// TwinCAT 3 PLC project TC3_SortingSystem_Simu
// libraries:
//   Tc2_Standard, * (Beckhoff Automation GmbH)
//   Tc2_System, * (Beckhoff Automation GmbH)
//   Tc3_Interfaces, * (Beckhoff Automation GmbH)
//   Tc3_Module, * (Beckhoff Automation GmbH)
// project tree:
//   / PlcTask_Simu.TcTTO, Visualization Manager.TcVMO
//   POUs/ MAIN_Simu.TcPOU
// real-time tasks:
//   TASK PlcTask: cycle T#10ms, priority 20, ADS port 350
//   TASK PlcTask_Simu: cycle T#10ms, priority 21, ADS port 351
// motion (NC):
//   TASK NC-Task 1 SAF: cycle T#2ms, priority 4, ADS port 501
//   TASK NC-Task 1 SVB: cycle T#10ms, priority 8, ADS port 511
//   AXIS Axis MetalSorting (id 1)
//     OtherSettings: AllowMotionCmdToSlave=true
//     encoder EncType=1
//     drive DrvType=5
//       TimeComp: TaskDelayCycles=1
//     controller CtrType=1
//       CtrPara: PriorControlFactor=1
//         Observer: BandWidth=20
//   AXIS Axis PlasticSorting (id 2)
//     OtherSettings: AllowMotionCmdToSlave=true
//     encoder EncType=1
//     drive DrvType=5
//     controller CtrType=1
//       CtrPara: PriorControlFactor=1
//         Observer: BandWidth=20
//   AXIS Axis Separating (id 3)
//     OtherSettings: AllowMotionCmdToSlave=true
//     encoder EncType=1
//     drive DrvType=5
//       TimeComp: TaskDelayCycles=1
//     controller CtrType=1
//       CtrPara: PriorControlFactor=1
//         Observer: BandWidth=20
// variable links:
//   TC3_SortingSystem_PLC/TC3_SortingSystem_PLC Instance <-> NC-Task 1 SAF/Axes/Axis MetalSorting
//     PlcTask Outputs/MAIN.fbMetalSorting.fbAxis.AxisRef.PlcToNc <-> Inputs/Axis MetalSorting_FromPlc
//     PlcTask Inputs/MAIN.fbMetalSorting.fbAxis.AxisRef.NcToPlc <-> Outputs/Axis MetalSorting_ToPlc
//   TC3_SortingSystem_PLC/TC3_SortingSystem_PLC Instance <-> NC-Task 1 SAF/Axes/Axis PlasticSorting
//     PlcTask Outputs/MAIN.fbPlasticSorting.fbAxis.AxisRef.PlcToNc <-> Inputs/Axis PlasticSorting_FromPlc
//     PlcTask Inputs/MAIN.fbPlasticSorting.fbAxis.AxisRef.NcToPlc <-> Outputs/Axis PlasticSorting_ToPlc
//   TC3_SortingSystem_PLC/TC3_SortingSystem_PLC Instance <-> NC-Task 1 SAF/Axes/Axis Separating
//     PlcTask Outputs/MAIN.fbSeparateModule.fbAxis.AxisRef.PlcToNc <-> Inputs/Axis Separating_FromPlc
//     PlcTask Inputs/MAIN.fbSeparateModule.fbAxis.AxisRef.NcToPlc <-> Outputs/Axis Separating_ToPlc
//   TC3_SortingSystem_PLC/TC3_SortingSystem_PLC Instance <-> TC3_SortingSystem_Simu/TC3_SortingSystem_Simu Instance
//     PlcTask Inputs/MAIN.fbSeparateModule.fbClampTemp.lrTempCurrent <-> PlcTask_Simu Outputs/MAIN_Simu.lrClampTempCurrent
//     PlcTask Inputs/MAIN.fbSeparateModule.fbClampTempDiag.bAtWorkPos <-> PlcTask_Simu Outputs/MAIN_Simu.bClampAtWork
//     PlcTask Inputs/MAIN.fbSeparateModule.fbClampTempDiag.lrTempMax <-> PlcTask_Simu Outputs/MAIN_Simu.lrClampTempMax
//     PlcTask Inputs/MAIN.fbSeparateModule.fbClampTempRecord.bAtBasePos <-> PlcTask_Simu Outputs/MAIN_Simu.bClampAtBase
//     PlcTask Inputs/MAIN.fbSeparateModule.fbClampTempRecord.lrTempCurrent <-> PlcTask_Simu Outputs/MAIN_Simu.lrClampTempCurrent
//     PlcTask Inputs/MAIN.fbSeparateModule.fbBarrier.bAtWorkPos <-> PlcTask_Simu Outputs/MAIN_Simu.bBarrierAtWork
//     PlcTask Inputs/MAIN.fbSeparateModule.fbBarrierDiag.bAtWorkPos <-> PlcTask_Simu Outputs/MAIN_Simu.bBarrierAtWork
//     PlcTask Inputs/MAIN.fbSeparateModule.fbBarrierTemp.bAtWorkPos <-> PlcTask_Simu Outputs/MAIN_Simu.bBarrierAtWork
//     PlcTask Inputs/MAIN.fbSeparateModule.fbBarrierTempDiag.bAtBasePos <-> PlcTask_Simu Outputs/MAIN_Simu.bBarrierAtBase
//     PlcTask Inputs/MAIN.fbSeparateModule.fbBarrierTempDiag.lrTempCurrent <-> PlcTask_Simu Outputs/MAIN_Simu.lrBarrierTemp
//     PlcTask Inputs/MAIN.fbMetalSorting.fbCylinder.bAtBasePos <-> PlcTask_Simu Outputs/MAIN_Simu.bMetalAtBase
//     PlcTask Inputs/MAIN.fbMetalSorting.fbCylinderDiag.bAtBasePos <-> PlcTask_Simu Outputs/MAIN_Simu.bMetalAtBase
//     PlcTask Inputs/MAIN.fbSeparateModule.fbBarrierTempRecord.bAtWorkPos <-> PlcTask_Simu Outputs/MAIN_Simu.bBarrierAtWork
//     PlcTask Inputs/MAIN.fbMetalSorting.fbCylinderTemp.bAtBasePos <-> PlcTask_Simu Outputs/MAIN_Simu.bMetalAtBase
//     PlcTask Outputs/MAIN.fbVisu.lrYClamp <-> PlcTask_Simu Inputs/MAIN_Simu.lrYClamp
//     PlcTask Outputs/MAIN.fbVisu.lrYBarrier <-> PlcTask_Simu Inputs/MAIN_Simu.lrYBarrier
//     PlcTask Outputs/MAIN.fbVisu.lrYMetal <-> PlcTask_Simu Inputs/MAIN_Simu.lrYMetal
//     PlcTask Outputs/MAIN.fbVisu.lrYPlastic <-> PlcTask_Simu Inputs/MAIN_Simu.lrYPlastic
//     PlcTask Inputs/MAIN.fbMetalSorting.fbCylinderTempDiag.bAtWorkPos <-> PlcTask_Simu Outputs/MAIN_Simu.bMetalAtWork
//     PlcTask Outputs/MAIN.fbVisu.lrBoxX <-> PlcTask_Simu Inputs/MAIN_Simu.lrBoxX
//     PlcTask Inputs/MAIN.fbPlasticSorting.fbSensorDelay.bInput <-> PlcTask_Simu Outputs/MAIN_Simu.bPlasticSensor
//     PlcTask Inputs/MAIN.fbPlasticSorting.fbCylinder.bAtWorkPos <-> PlcTask_Simu Outputs/MAIN_Simu.bPlasticAtWork
//     PlcTask Inputs/MAIN.fbMetalSorting.fbCylinderTempRecord.bAtBasePos <-> PlcTask_Simu Outputs/MAIN_Simu.bMetalAtBase
//     PlcTask Inputs/MAIN.fbPlasticSorting.fbCylinderDiag.bAtWorkPos <-> PlcTask_Simu Outputs/MAIN_Simu.bPlasticAtWork
//     PlcTask Outputs/MAIN.fbVisu.lrBoxY <-> PlcTask_Simu Inputs/MAIN_Simu.lrBoxY
//     PlcTask Inputs/MAIN.fbPlasticSorting.fbCylinderTemp.bAtWorkPos <-> PlcTask_Simu Outputs/MAIN_Simu.bPlasticAtWork
//     PlcTask Inputs/MAIN.fbPlasticSorting.fbCylinderTempDiag.bAtBasePos <-> PlcTask_Simu Outputs/MAIN_Simu.bPlasticAtBase
//     PlcTask Inputs/MAIN.fbSeparateModule.fbClamp.bAtBasePos <-> PlcTask_Simu Outputs/MAIN_Simu.bClampAtBase
//     PlcTask Inputs/MAIN.fbSeparateModule.fbClampDiag.bAtBasePos <-> PlcTask_Simu Outputs/MAIN_Simu.bClampAtBase
//     PlcTask Inputs/MAIN.fbSeparateModule.fbClampTemp.bAtBasePos <-> PlcTask_Simu Outputs/MAIN_Simu.bClampAtBase
//     PlcTask Inputs/MAIN.fbSeparateModule.fbClampTempDiag.bAtBasePos <-> PlcTask_Simu Outputs/MAIN_Simu.bClampAtBase
//     PlcTask Inputs/MAIN.fbSeparateModule.fbBarrier.bAtBasePos <-> PlcTask_Simu Outputs/MAIN_Simu.bBarrierAtBase
//     PlcTask Inputs/MAIN.fbSeparateModule.fbBarrierDiag.bAtBasePos <-> PlcTask_Simu Outputs/MAIN_Simu.bBarrierAtBase
//     PlcTask Inputs/MAIN.fbSeparateModule.fbBarrierTemp.bAtBasePos <-> PlcTask_Simu Outputs/MAIN_Simu.bBarrierAtBase
//     PlcTask Inputs/MAIN.fbSeparateModule.fbBarrierTempRecord.bAtBasePos <-> PlcTask_Simu Outputs/MAIN_Simu.bBarrierAtBase
//     PlcTask Inputs/MAIN.fbMetalSorting.fbCylinderTempDiag.bAtBasePos <-> PlcTask_Simu Outputs/MAIN_Simu.bMetalAtBase
//     PlcTask Inputs/MAIN.fbPlasticSorting.fbCylinderTempRecord.bAtWorkPos <-> PlcTask_Simu Outputs/MAIN_Simu.bPlasticAtWork
//     PlcTask Inputs/MAIN.fbPlasticSorting.fbCylinder.bAtBasePos <-> PlcTask_Simu Outputs/MAIN_Simu.bPlasticAtBase
//     PlcTask Inputs/MAIN.fbPlasticSorting.fbCylinderDiag.bAtBasePos <-> PlcTask_Simu Outputs/MAIN_Simu.bPlasticAtBase
//     PlcTask Inputs/MAIN.fbPlasticSorting.fbCylinderTemp.bAtBasePos <-> PlcTask_Simu Outputs/MAIN_Simu.bPlasticAtBase
//     PlcTask Inputs/MAIN.fbPlasticSorting.fbCylinderTempRecord.bAtBasePos <-> PlcTask_Simu Outputs/MAIN_Simu.bPlasticAtBase
//     PlcTask Inputs/MAIN.fbVisu.bBarrierSensor <-> PlcTask_Simu Outputs/MAIN_Simu.bBarrierSensor
//     PlcTask Inputs/MAIN.fbSeparateModule.fbSensor.bInput <-> PlcTask_Simu Outputs/MAIN_Simu.bBarrierSensor
//     PlcTask Inputs/MAIN.fbVisu.bPlasticSensor <-> PlcTask_Simu Outputs/MAIN_Simu.bPlasticSensor
//     PlcTask Inputs/MAIN.fbSeparateModule.fbClamp.bAtWorkPos <-> PlcTask_Simu Outputs/MAIN_Simu.bClampAtWork
//     PlcTask Inputs/MAIN.fbSeparateModule.fbClampDiag.bAtWorkPos <-> PlcTask_Simu Outputs/MAIN_Simu.bClampAtWork
//     PlcTask Inputs/MAIN.fbSeparateModule.fbBarrierTemp.lrTempCurrent <-> PlcTask_Simu Outputs/MAIN_Simu.lrBarrierTemp
//     PlcTask Inputs/MAIN.fbSeparateModule.fbBarrierTempRecord.lrTempCurrent <-> PlcTask_Simu Outputs/MAIN_Simu.lrBarrierTemp
//     PlcTask Inputs/MAIN.fbSeparateModule.fbClampTemp.bAtWorkPos <-> PlcTask_Simu Outputs/MAIN_Simu.bClampAtWork
//     PlcTask Inputs/MAIN.fbSeparateModule.fbClampTempDiag.lrTempCurrent <-> PlcTask_Simu Outputs/MAIN_Simu.lrClampTempCurrent
//     PlcTask Inputs/MAIN.fbSeparateModule.fbClampTempDiag.lrTempMin <-> PlcTask_Simu Outputs/MAIN_Simu.lrClampTempMin
//     PlcTask Inputs/MAIN.fbSeparateModule.fbClampTempRecord.bAtWorkPos <-> PlcTask_Simu Outputs/MAIN_Simu.bClampAtWork
//     PlcTask Inputs/MAIN.fbSeparateModule.fbBarrierTempDiag.bAtWorkPos <-> PlcTask_Simu Outputs/MAIN_Simu.bBarrierAtWork
//     PlcTask Inputs/MAIN.fbMetalSorting.fbSensorDelay.bInput <-> PlcTask_Simu Outputs/MAIN_Simu.bMetalSensor
//     PlcTask Inputs/MAIN.fbMetalSorting.fbCylinder.bAtWorkPos <-> PlcTask_Simu Outputs/MAIN_Simu.bMetalAtWork
//     PlcTask Inputs/MAIN.fbMetalSorting.fbCylinderDiag.bAtWorkPos <-> PlcTask_Simu Outputs/MAIN_Simu.bMetalAtWork
//     PlcTask Outputs/MAIN.bReset <-> PlcTask_Simu Inputs/MAIN_Simu.bReset
//     PlcTask Inputs/MAIN.fbMetalSorting.fbCylinderTemp.bAtWorkPos <-> PlcTask_Simu Outputs/MAIN_Simu.bMetalAtWork
//     PlcTask Inputs/MAIN.fbMetalSorting.fbCylinderTempRecord.bAtWorkPos <-> PlcTask_Simu Outputs/MAIN_Simu.bMetalAtWork
//     PlcTask Inputs/MAIN.fbPlasticSorting.fbCylinderTempDiag.bAtWorkPos <-> PlcTask_Simu Outputs/MAIN_Simu.bPlasticAtWork
//     PlcTask Inputs/MAIN.fbVisu.bMetalSensor <-> PlcTask_Simu Outputs/MAIN_Simu.bMetalSensor

CONFIGURATION TC3_SortingSystem_Simu
    RESOURCE PLC ON TwinCAT3
        TASK PlcTask_Simu(INTERVAL := T#10ms, PRIORITY := 21);
        PROGRAM MAIN_Simu WITH PlcTask_Simu : MAIN_Simu;
    END_RESOURCE
END_CONFIGURATION

// ---- POUs/MAIN_Simu.TcPOU
PROGRAM MAIN_Simu
VAR
	bReset						AT %I*: BOOL;
(***** Cylinder states *****)
	bClampAtBase				AT %Q*: BOOL;			// True if clamp cylinder is in base position
	bClampAtWork				AT %Q*: BOOL;			// True if clamp cylinder is in work position
	bBarrierAtBase				AT %Q*: BOOL;			// True if barrier cylinder is in base position
	bBarrierAtWork				AT %Q*: BOOL;			// True if barrier cylinder is in work position
	bMetalAtBase				AT %Q*: BOOL;			// True if metal cylinder is in base position
	bMetalAtWork				AT %Q*: BOOL;			// True if metal cylinder is in work position
	bPlasticAtBase				AT %Q*: BOOL;			// True if plastic cylinder is in base position
	bPlasticAtWork				AT %Q*: BOOL;			// True if plastic cylinder is in work position
(***** Temperatures *****)
	lrClampTempCurrent			AT %Q*: LREAL;			// Current temperature of clamp cylinder
	lrClampTempMax				AT %Q*: LREAL;			// Maximum temperature of clamp cylinder
	lrClampTempMin				AT %Q*: LREAL;			// Minimum temperature of clamp cylinder
	lrBarrierTemp				AT %Q*: LREAL;			// Temperature of barrier cylinder

(***** Sensors to detect boxes *****)
	bBarrierSensor				AT %Q*: BOOL;			// True if barrier sensor detects a box
	bMetalSensor				AT %Q*: BOOL;			// True if metal sensor detects a metal box
	bPlasticSensor				AT %Q*: BOOL;			// True if plastic sensor detects a box

(* Position variables *)
	lrYClamp					AT %I*: LREAL;					// Y-Coordinate of clamp cylinder
	lrYBarrier					AT %I*: LREAL;					// Y-Coordinate of barrier cylinder
	lrYMetal					AT %I*: LREAL;					// Y-Coordinate of metal cylinder
	lrYPlastic					AT %I*: LREAL;					// Y-Coordinate of plastic cylinder
	lrBoxX						AT %I*: ARRAY[1..4] OF LREAL;	// X-Coordinates of boxes
	lrBoxY						AT %I*: ARRAY[1..4] OF LREAL;	// Y-Coordinates of boxes
	
	bTempUp						: BOOL;					// To raise temperature of clamp cylinder
	tonTemp						: TON;					// Timer to change temperature
END_VAR

// =========================================================
	// Resetting temperatures
	
IF bReset THEN
	lrClampTempCurrent := 0;
	lrBarrierTemp := 0;
END_IF

// =========================================================
	// Cylinder temperatures
	
A_Temperatures();

// =========================================================
	// Output variables
	
A_SetOutput();

// =========================================================

ACTION A_SetOutput:
// =========================================================
	// Cylinder variables
	
bClampAtWork := (lrYClamp = 3.0);
bClampAtBase := (lrYClamp = 0.0);
bBarrierAtWork := (lrYBarrier = 63.0);
bBarrierAtBase := (lrYBarrier = 0.0);
bMetalAtWork := (lrYMetal < -72.9) AND (lrYMetal > -73.1);
bMetalAtBase := (lrYMetal = 0.0);
bPlasticAtWork := (lrYPlastic < -72.9) AND (lrYPlastic > -73.1);
bPlasticAtBase := (lrYPlastic = 0.0);

// =========================================================
	// Sensor variables
	
bBarrierSensor := ( (lrBoxY[1] >= -5) AND (lrBoxX[1] > -1) AND (lrBoxX[1] < 60) )
				OR ( (lrBoxY[2] >= -5) AND (lrBoxX[2] > 59) AND (lrBoxX[2] < 120) )
				OR ( (lrBoxY[3] >= -5) AND (lrBoxX[3] > 119) AND (lrBoxX[3] < 180) )
				OR ( (lrBoxY[4] >= -5) AND (lrBoxX[4] > 179) AND (lrBoxX[4] < 240) );
				
bMetalSensor := ( (lrBoxY[1] >= -5) AND (lrBoxX[1] > 134) AND (lrBoxX[1] < 197) )
				OR ( (lrBoxY[4] >= -5) AND (lrBoxX[4] > 314) AND (lrBoxX[4] < 377) );
				
bPlasticSensor := ( (lrBoxY[1] >= -5) AND (lrBoxX[1] > 384) AND (lrBoxX[1] < 447) )
				OR ( (lrBoxY[2] >= -5) AND (lrBoxX[2] > 444) AND (lrBoxX[2] < 507) )
				OR ( (lrBoxY[3] >= -5) AND (lrBoxX[3] > 504) AND (lrBoxX[3] < 567) )
				OR ( (lrBoxY[4] >= -5) AND (lrBoxX[4] > 564) AND (lrBoxX[4] < 627) );

// =========================================================
END_ACTION

ACTION A_Temperatures:
// =========================================================
	// Temperature of cylinders
	
lrClampTempMax := 60.5;
lrClampTempMin := 9.4;
lrClampTempCurrent := 10.7;

tonTemp( PT := T#1S );
IF NOT tonTemp.Q THEN
	tonTemp( IN := TRUE );
END_IF

IF lrBarrierTemp >= 55 THEN
	bTempUp := FALSE;
ELSIF lrBarrierTemp <=	10 THEN
	bTempUp := TRUE;
END_IF

IF tonTemp.Q THEN
	tonTemp( IN := FALSE );
	IF bTempUp THEN
		lrBarrierTemp := lrBarrierTemp + 1.2;
	ELSE
		lrBarrierTemp := lrBarrierTemp - 1.2;
	END_IF
END_IF

// =========================================================
END_ACTION

END_PROGRAM
